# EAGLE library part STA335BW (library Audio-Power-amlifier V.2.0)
The STA335BW is an integration of digital audio processing, digital amplifier control and DDX® power-output stage to create a high-power single-chip DDX solution comprising high-quality, high-efficiency and all digital amplification. The STA335BW is part of the Sound Terminal™ family that provides full digital audio streaming to the speaker offering cost effectiveness, low energy dissipation and sound enrichment. The STA335BW power section consists of four independent half-bridges. These can be configured via digital control to operate in different modes. 2.1 channels can be provided by two half-bridges and a single full-bridge, providing up to 2 x 9 W + 1 x 20 W of power output. Two channels can be provided by two full-bridges, providing up to 2 x 37 W of power. The IC can also be configured as 2.1 channels with 2 x 30 W provided by the device and external power for DDX® power drive.
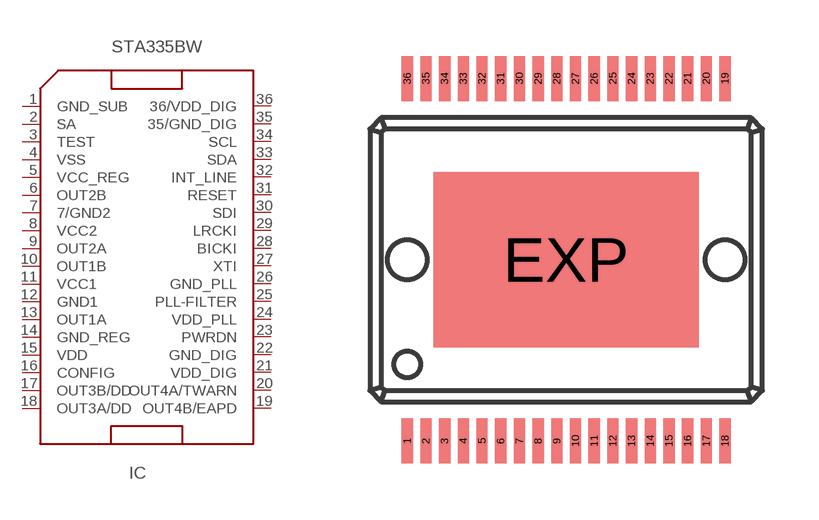
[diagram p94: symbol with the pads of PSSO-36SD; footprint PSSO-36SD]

Designator prefix IC

## STA335BW  [PSSO-36SD]
1  GND_SUB  pwr
2  SA  in
3  TEST  in
4  VSS
5  VCC_REG
6  OUT2B  out
7  7/GND2  pwr
8  VCC2  pwr
9  OUT2A  out
10  OUT1B  out
11  VCC1  pwr
12  GND1  pwr
13  OUT1A
14  GND_REG  pwr
15  VDD  pwr
16  CONFIG  in
17  OUT3B/DD  out
18  OUT3A/DD  out
19  OUT4B/EAPD  out
20  OUT4A/TWARN  in
21  VDD_DIG  pwr
22  GND_DIG  pwr
23  PWRDN  in
24  VDD_PLL  pwr
25  PLL-FILTER  in
26  GND_PLL  pwr
27  XTI  in
28  BICKI  in
29  LRCKI  in
30  SDI  in
31  RESET  in
32  INT_LINE  out
33  SDA
34  SCL  in
35  35/GND_DIG  pwr
36  36/VDD_DIG  pwr

## Footprint PSSO-36SD (pad centres in mm)
PowerSSO-36 slug down package
smd 0.3 x 1.2: 1 -4.25,-4.85; 2 -3.75,-4.85; 3 -3.25,-4.85; 4 -2.75,-4.85; 5 -2.25,-4.85; 6 -1.75,-4.85; 7 -1.25,-4.85; 8 -0.75,-4.85; 9 -0.25,-4.85; 10 0.25,-4.85; 11 0.75,-4.85; 12 1.25,-4.85; 13 1.75,-4.85; 14 2.25,-4.85; 15 2.75,-4.85; 16 3.25,-4.85; 17 3.75,-4.85; 18 4.25,-4.85; 19 4.25,4.85; 20 3.75,4.85; 21 3.25,4.85; 22 2.75,4.85; 23 2.25,4.85; 24 1.75,4.85; 25 1.25,4.85; 26 0.75,4.85; 27 0.25,4.85; 28 -0.25,4.85; 29 -0.75,4.85; 30 -1.25,4.85; 31 -1.75,4.85; 32 -2.25,4.85; 33 -2.75,4.85; 34 -3.25,4.85; 35 -3.75,4.85; 36 -4.25,4.85
smd 7.1 x 4.7: EXP 0,0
